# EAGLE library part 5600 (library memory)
MEMORY
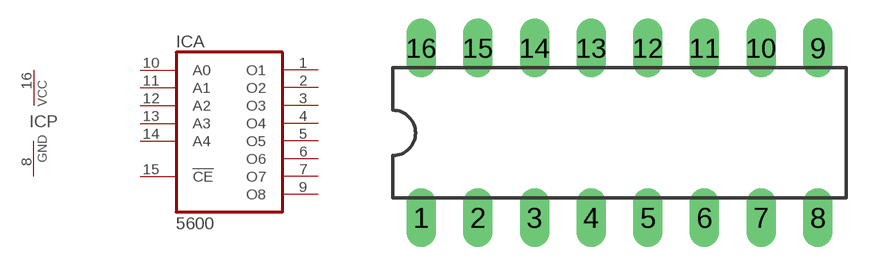
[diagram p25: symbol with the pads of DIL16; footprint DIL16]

Designator prefix IC; gates A=5600 P=PWRN

## 5600  [DIL16]
1  A:O1  oc
2  A:O2  oc
3  A:O3  oc
4  A:O4  oc
5  A:O5  oc
6  A:O6  oc
7  A:O7  oc
8  P:GND  pwr
9  A:O8  oc
10  A:A0  in
11  A:A1  in
12  A:A2  in
13  A:A3  in
14  A:A4  in
15  A:!CE  in
16  P:VCC  pwr

## Footprint DIL16 (pad centres in mm)
Dual In Line Package
drill 0.813 long: 1 -8.89,-3.81; 2 -6.35,-3.81; 3 -3.81,-3.81; 4 -1.27,-3.81; 5 1.27,-3.81; 6 3.81,-3.81; 7 6.35,-3.81; 8 8.89,-3.81; 9 8.89,3.81; 10 6.35,3.81; 11 3.81,3.81; 12 1.27,3.81; 13 -1.27,3.81; 14 -3.81,3.81; 15 -6.35,3.81; 16 -8.89,3.81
